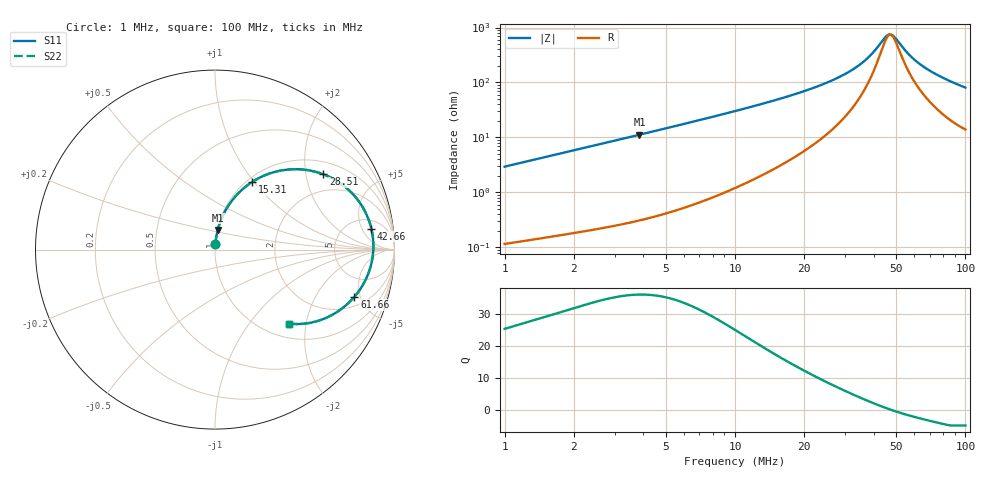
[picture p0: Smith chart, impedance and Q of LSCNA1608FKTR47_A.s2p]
! LSCNA1608FKTR47_A  S-PARAMETER MODEL  ( Standard Model )
! Model Generated by TAIYO YUDEN Corporation (http://www.ty-top.com)
! Version 1.0
! TAIYO YUDEN Control No. 160926
! Copyright(c) 2016 TAIYO YUDEN CO.,LTD. All Rights Reserved.
! Product Description (link to TY-COMPAS)
! https://ds.yuden.co.jp/TYCOMPAS/or/detail?pn=LSCNA1608FKTR47MA&u=M
! Products Name : Inductors
! Characteristics :
!  Inductance : 0.47 [uH] , SRF(min) : - [Hz] , DC Resistance(max) : 85 [mOhm]
!  Rated Current : Saturation  1.9 [A] (dL = 30 [%]), Temp Rise  1.6 [A] (dT = 40 [degC])
!  Case Size : 1.6 x 0.8 / 0.063 x 0.031 [mm/inch] , Thickness : 0.6 / 0.024 [mm/inch]
!  (Conditions: Temperature = 25 [degC] , DC Bias Current = 0 [A])
! External Node Assignments :
!  1  o---GGG---o  2
! GND o---------o GND
! Frequency Range : 1MHz  -  100MHz  [ 402 STEP ]
# MHz S RI R 50
! Freq[MHz].  S11 Real  S11 Imag  S21 Real  S21 Imag  S12 Real  S12 Imag  S22 Real  S22 Imag
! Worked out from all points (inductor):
!   401 points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, 1 MHz to 100 MHz, reference 50 ohm
!   read as one part in series: L = 466 nH near 1.023 MHz
!   highest Q = 36.3 at 3.846 MHz (marker M1), where L = 463 nH
!   self-resonance near 47.26 MHz
!   S11 on the Smith chart (normalised r, x): 1 MHz: 1.00, +0.06; 15.31 MHz: 1.06, +0.98; 28.51 MHz: 1.38, +2.51; 42.66 MHz: 8, +8; 61.66 MHz: 2.75, -4.41; 100 MHz: 1.28, -1.59
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1  0.00201 0.0293  0.998 -0.0293  0.998 -0.0293  0.00201 0.0293
1.496236  0.00339 0.0435  0.9966 -0.0435  0.9966 -0.0435  0.00339 0.0435
2.113489  0.00564 0.0611  0.9944 -0.0611  0.9944 -0.0611  0.00564 0.0611
3.845918  0.0153 0.1098  0.9847 -0.1098  0.9847 -0.1098  0.0153 0.1098
5.821032  0.0328 0.164  0.9672 -0.164  0.9672 -0.164  0.0328 0.164
8.317638  0.0647 0.2291  0.9353 -0.2291  0.9353 -0.2291  0.0647 0.2291
15.31087  0.208 0.3774  0.792 -0.3774  0.792 -0.3774  0.208 0.3774
17.57924  0.269 0.4102  0.731 -0.4102  0.731 -0.4102  0.269 0.4102
23.17395  0.4378 0.4479  0.5622 -0.4479  0.5622 -0.4479  0.4378 0.4479
28.51018  0.6028 0.42  0.3972 -0.42  0.3972 -0.42  0.6028 0.42
34.27678  0.7533 0.3246  0.2467 -0.3246  0.2467 -0.3246  0.7533 0.3246
38.45918  0.8288 0.226  0.1712 -0.226  0.1712 -0.226  0.8288 0.226
42.65795  0.8712 0.1169  0.1288 -0.1169  0.1288 -0.1169  0.8712 0.1169
45.18559  0.8813 0.0515  0.1187 -0.0515  0.1187 -0.0515  0.8813 0.0515
46.77351  0.8825 0.0119  0.1175 -0.0119  0.1175 -0.0119  0.8825 0.0119
48.41724  0.88 -0.0275  0.12 0.0275  0.12 0.0275  0.88 -0.0275
50.69907  0.871 -0.0789  0.129 0.0789  0.129 0.0789  0.871 -0.0789
56.23413  0.8306 -0.1848  0.1694 0.1848  0.1694 0.1848  0.8306 -0.1848
61.6595  0.7764 -0.2634  0.2236 0.2634  0.2236 0.2634  0.7764 -0.2634
67.6083  0.7113 -0.3252  0.2887 0.3252  0.2887 0.3252  0.7113 -0.3252
84.13951  0.5388 -0.4062  0.4612 0.4062  0.4612 0.4062  0.5388 -0.4062
100  0.4098 -0.4118  0.5902 0.4118  0.5902 0.4118  0.4098 -0.4118
